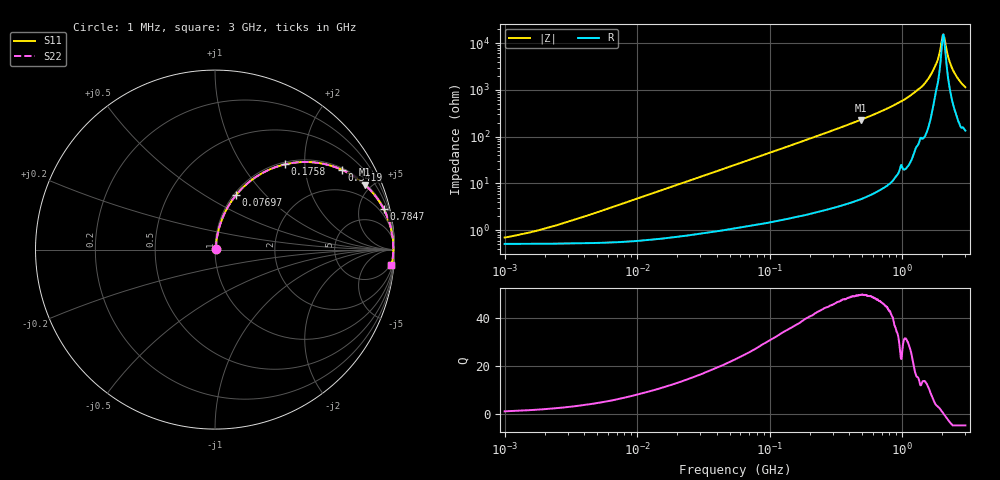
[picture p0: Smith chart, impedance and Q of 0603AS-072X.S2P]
!s-Parameter Generated by FASTRON Sdn. Bhd.
!FASTRON P/N : 0603AS-072X
!Keysight Technologies: E4991B_MY54100416_A.01.15
!Date created: Tue Oct 17 15:58:06 2023
!Version  : Rev01 Tue Oct 17 15:58:06 2023
!Data & Calibration Information:
!Freq	S11	S21	S12	S22
!PortZ  Port1:50+j0  Port2:50+j0
!When reading reference impedance value at option line is always used.
! Remarks : This data is being provided solely for informational purposes.
# Hz S dB R 50
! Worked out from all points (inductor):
!   1601 points, 1 MHz to 3 GHz, reference 50 ohm
!   read as one part in series: L = 75.2 nH near 3.307 MHz
!   highest Q = 49.8 at 485.4 MHz (marker M1), where L = 74.8 nH
!   self-resonance near 2.041 GHz
!   S11 on the Smith chart (normalised r, x): 1 MHz: 1.01, +0.01; 76.97 MHz: 1.03, +0.70; 175.8 MHz: 1.04, +1.58; 341.9 MHz: 1.07, +3.13; 784.7 MHz: 1.19, +8.18; 3 GHz: 4, -23
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1000000  -43.17 42.8  -0.04 -0.3  -0.04 -0.3  -43.17 42.8
3804036  -34.60 72.7  -0.05 -1.0  -0.05 -1.0  -34.60 72.7
1.447069e7  -23.46 80.7  -0.08 -3.8  -0.08 -3.8  -23.46 80.7
5.477226e7  -12.41 73.6  -0.35 -13.9  -0.35 -13.9  -12.41 73.6
7.697298e7  -9.74 68.9  -0.60 -19.0  -0.60 -19.0  -9.74 68.9
1.757585e8  -4.24 50.7  -2.22 -37.8  -2.22 -37.8  -4.24 50.7
2.083556e8  -3.39 46.0  -2.86 -42.6  -2.86 -42.6  -3.39 46.0
3.419417e8  -1.57 32.2  -5.46 -56.6  -5.46 -56.6  -1.57 32.2
4.853736e8  -0.83 23.5  -8.00 -65.4  -8.00 -65.4  -0.83 23.5
7.846996e8  -0.30 13.7  -12.54 -75.0  -12.54 -75.0  -0.30 13.7
7.925923e8  -0.29 13.5  -12.65 -75.2  -12.65 -75.2  -0.29 13.5
1.113852e9  -0.13 8.0  -17.12 -80.0  -17.12 -80.0  -0.13 8.0
1.503902e9  -0.07 3.9  -23.30 -81.7  -23.30 -81.7  -0.07 3.9
1.800756e9  -0.07 1.6  -31.03 -73.0  -31.03 -73.0  -0.07 1.6
1.883708e9  -0.06 1.0  -34.19 -68.1  -34.19 -68.1  -0.06 1.0
1.990301e9  -0.06 0.3  -41.11 -42.5  -41.11 -42.5  -0.06 0.3
2.040726e9  -0.06 0.0  -43.75 -3.6  -43.75 -3.6  -0.06 0.0
2.092429e9  -0.06 -0.3  -41.62 37.6  -41.62 37.6  -0.06 -0.3
2.255531e9  -0.06 -1.2  -32.94 71.2  -32.94 71.2  -0.06 -1.2
2.407135e9  -0.07 -2.1  -28.76 76.8  -28.76 76.8  -0.07 -2.1
2.714296e9  -0.08 -3.6  -23.94 79.7  -23.94 79.7  -0.08 -3.6
3e9  -0.12 -4.9  -21.29 78.3  -21.29 78.3  -0.12 -4.9
